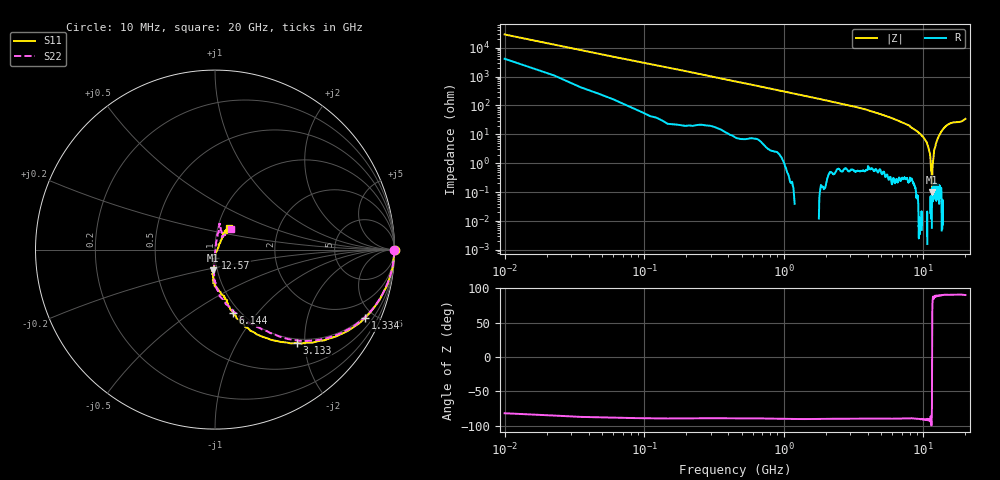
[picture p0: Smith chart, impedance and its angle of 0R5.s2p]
!Keysight Technologies,P5008B,MY61100088,A.16.20.02
!Date: Monday, May 27, 2024 13:23:29
!Correction: S11(C  2-Port  )
!S21(C  2-Port  )
!S12(C  2-Port  )
!S22(C  2-Port  )
!S2P File: Measurements: S11, S21, S12, S22:
# Hz S  dB  R 50
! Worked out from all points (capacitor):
!   1601 points, 10 MHz to 20 GHz, reference 50 ohm
!   read as one part in series: C = 523 fF near 110 MHz
!   lowest |Z| = 102 mohm at 11.54 GHz (marker M1)
!   series resonance near 11.55 GHz, so ESL is about 360 pH
!   S11 on the Smith chart (normalised r, x): 10 MHz: open; 1.334 GHz: 0.91, -4.42; 3.133 GHz: 0.92, -1.83; 6.144 GHz: 0.93, -0.75; 12.57 GHz: 1.00, -0.09; 20 GHz: 1.13, +0.27
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1e7  0.01 -0.2  -49.13 81.5  -49.44 82.3  -0.01 -0.2
1.474312e8  -0.03 -2.9  -26.29 86.5  -26.29 86.5  -0.02 -2.8
3.473312e8  -0.07 -6.7  -18.91 82.4  -18.92 82.4  -0.07 -6.6
7.221438e8  -0.26 -13.6  -12.85 75.9  -12.86 76.0  -0.25 -13.3
1.334338e9  -0.74 -24.5  -7.99 66.1  -8.00 66.1  -0.72 -23.7
3.133438e9  -3.21 -48.9  -2.80 41.4  -2.81 41.4  -3.20 -47.2
3.345831e9  -3.53 -51.5  -2.51 39.1  -2.52 39.1  -3.56 -49.2
6.144431e9  -8.74 -74.2  -0.61 15.7  -0.62 15.8  -8.73 -72.6
6.681662e9  -9.70 -75.9  -0.47 12.7  -0.49 12.7  -9.69 -76.5
1.0005e10  -14.60 -92.9  -0.11 -1.8  -0.13 -1.7  -14.65 -88.8
1.154173e10  -18.71 -94.8  -0.02 -6.7  -0.03 -6.7  -18.51 -92.7
1.256622e10  -26.93 -90.0  0.03 -10.1  0.02 -10.0  -26.73 -91.4
1.295352e10  -35.57 -73.6  0.04 -11.4  0.03 -11.4  -36.06 -90.3
1.314093e10  -38.17 -19.4  0.04 -12.0  0.03 -11.9  -50.41 -24.7
1.322839e10  -36.80 10.5  0.04 -12.3  0.03 -12.2  -43.14 86.8
1.334083e10  -33.13 30.9  0.05 -12.6  0.04 -12.6  -36.12 84.8
1.349076e10  -29.29 54.2  0.04 -13.2  0.03 -13.1  -30.00 77.5
1.377811e10  -25.13 56.0  0.06 -14.1  0.05 -14.1  -25.68 79.8
1.441529e10  -19.96 62.6  0.03 -16.4  0.02 -16.4  -20.18 78.3
1.667666e10  -17.25 54.1  -0.00 -22.6  -0.01 -22.6  -17.31 78.1
1.861319e10  -21.95 59.5  0.05 -28.1  0.04 -28.0  -21.75 61.0
2e10  -17.00 56.9  -0.02 -32.7  -0.03 -32.7  -16.81 53.2
